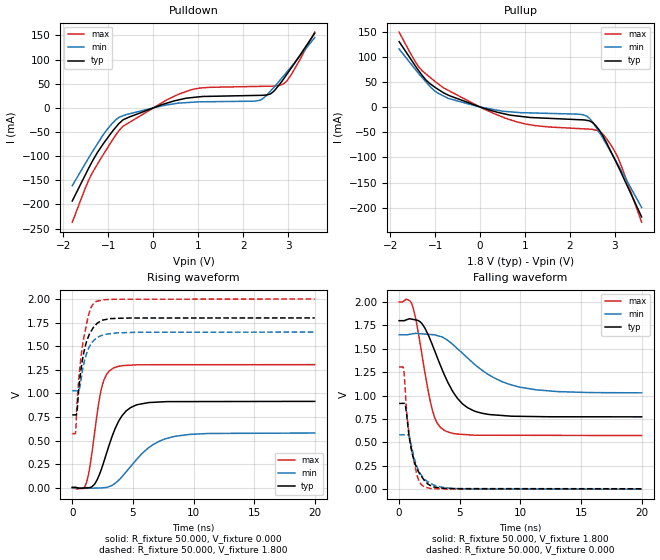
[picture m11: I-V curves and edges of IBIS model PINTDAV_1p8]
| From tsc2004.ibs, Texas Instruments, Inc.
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| Model 1.8 V PINTDAV
[Model]   PINTDAV_1p8
Model_type  Output
Polarity   Non-Inverting
Enable   Active-Low
Vmeas = 0.9
Vref = 0.9
Cref = 15pF
Rref = 50
|   typ   min   max
|   (nom PVT)   (Fast PVT)   (slow PVT)
|   Output High
C_comp   8.87322E-12   8.67118E-12   8.99669E-12
|   Output Low
|C_comp   8.83242E-12   8.51294E-12   9.03821E-12
| Where   nom PVT is  Nominal Process, 3.3V, 25C
|   Fast PVT is Strong Process, 3.6V, -40C
|   Slow PVT is Weak Process, 3.0V, 85C
|C_comp - from L-C Tank method, L = 1nH, peak frequency ~ 1.7GHz
[Voltage Range]   1.8   1.65   2
[Temperature Range]   30   88   -40
|Ambient Temperature Range 27   85   -40
[Pullup Reference]   1.8   1.65   2
[Pulldown Reference]   0   0   0
[Power Clamp Reference]   1.8   1.65   2
[GND Clamp Reference]   0   0   0
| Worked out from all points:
|   slope of the pulldown table from 0 to 0.27 V, typ, clamps not added: 30 ohm
|   slope of the pullup table from 0 to 0.27 V, typ, clamps not added: 35.3 ohm
|   falling waveform, R_fixture 50.000, V_fixture 1.800: 20-80 % time 2.19ns typ, 3.82ns min, 1.19ns max; typ from 1.8 V to 0.773 V
|   rising waveform, R_fixture 50.000, V_fixture 0.000: 20-80 % time 1.58ns typ, 2.67ns min, 896ps max; typ from 0.004 V to 0.915 V
|   rising waveform, R_fixture 50.000, V_fixture 1.800: 20-80 % time 817ps typ, 825ps min, 772ps max; typ from 0.773 V to 1.8 V
|   falling waveform, R_fixture 50.000, V_fixture 0.000: 20-80 % time 926ps typ, 1.03ns min, 772ps max; typ from 0.915 V to 0.004 V
[Pulldown]
|   Voltage   I(typ)   I(min)   I(max)
-1.8V     -192.8mA   -161.2mA   -236.8mA
-1.367V   -113.1mA   -93.03mA   -136.8mA
-929mV    -51.54mA   -34.05mA   -69.98mA
-672.1mV  -25.07mA   -16.42mA   -38.26mA
304.8mV   9.753mA    6.08mA     16.62mA
857.6mV   21.19mA    11.51mA    37.73mA
2.253V    25.62mA    13.81mA    44.22mA
2.436V    25.95mA    18.87mA    44.55mA
2.598V    28.47mA    33.64mA    44.83mA
2.8V      47.43mA    54.84mA    46.31mA
2.975V    69.69mA    74.32mA    55.61mA
3.595V    154.7mA    145.6mA    156.9mA
[Pullup]
|   Voltage   I(typ)   I(min)   I(max)
-1.8V     130mA      115.4mA    149.1mA
-1.281V   62.11mA    57.86mA    71.56mA
-1.017V   40.27mA    32.77mA    52.02mA
-704.3mV  23.56mA    17.18mA    33.06mA
24.07mV   -504.5uA   -278.9uA   -1.076mA
1.03V     -19.85mA   -11.4mA    -34.01mA
2.201V    -25.11mA   -14.15mA   -42.81mA
2.5V      -30.54mA   -29.5mA    -44.37mA
2.7V      -52.62mA   -57.02mA   -51.07mA
2.988V    -102.5mA   -101.6mA   -86.38mA
3.139V    -130.6mA   -125.7mA   -116.3mA
3.595V    -218.5mA   -199.7mA   -228.9mA
[Ramp]
R_load = 50
|   typ   min   max
dV/dt_r   0.561804/1.57452e-009  0.347932/2.64803e-009  0.782955/8.93072e-010
dV/dt_f   0.616385/2.18562e-009   0.37262/3.79469e-009  0.856164/1.19045e-009
[Falling Waveform]
R_fixture = 50.000
V_fixture = 1.800
V_fixture_min = 1.650
V_fixture_max = 2.000
C_fixture = 0.000
|  time   V(typ)   V(min)   V(max)
0s        1.8V       1.65V      2V
1.095ns   1.815V     1.659V     1.961V
1.91ns    1.764V     1.659V     1.413V
2.723ns   1.547V     1.651V     852.5mV
3.133ns   1.411V     1.641V     708.1mV
3.749ns   1.216V     1.611V     626.1mV
5.196ns   915.1mV    1.455V     585.3mV
6.838ns   810.9mV    1.271V     576.1mV
11.33ns   775.4mV    1.061V     575.1mV
20ns      772.7mV    1.029V     573.1mV
[Rising Waveform]
R_fixture = 50.000
V_fixture = 0.000
V_fixture_min = 0.000
V_fixture_max = 0.000
C_fixture = 0.000
|  time   V(typ)   V(min)   V(max)
0s        4.324mV    1.068uV    30.67nV
1.151ns   -1.527mV   -6.198mV   45.59mV
1.827ns   36.11mV    -4.034mV   568mV
2.411ns   200.4mV    -2.164mV   1.054V
2.816ns   361.1mV    3.376mV    1.199V
3.439ns   595.4mV    38.12mV    1.272V
4.804ns   849.1mV    223.4mV    1.299V
6.328ns   903mV      426.7mV    1.303V
8.303ns   912.9mV    540.5mV    1.304V
20ns      915.4mV    579.9mV    1.305V
[Rising Waveform]
R_fixture = 50.000
V_fixture = 1.800
V_fixture_min = 1.650
V_fixture_max = 2.000
C_fixture = 0.000
|  time   V(typ)   V(min)   V(max)
0s        772.7mV    1.029V     573.1mV
280.3ps   771.8mV    1.028V     597.8mV
398.1ps   814.7mV    1.027V     906.5mV
549.9ps   1.062V     1.036V     1.169V
739.7ps   1.273V     1.158V     1.408V
960.5ps   1.439V     1.319V     1.599V
1.471ns   1.642V     1.509V     1.885V
1.964ns   1.731V     1.583V     1.974V
4.572ns   1.799V     1.645V     1.999V
20ns      1.8V       1.65V      2V
[Falling Waveform]
R_fixture = 50.000
V_fixture = 0.000
V_fixture_min = 0.000
V_fixture_max = 0.000
C_fixture = 0.000
|  time   V(typ)   V(min)   V(max)
0s        915.4mV    579.9mV    1.305V
377ps     917mV      581.4mV    1.279V
548.5ps   868.7mV    582.1mV    956mV
763.5ps   626.6mV    574mV      649.5mV
1.045ns   400.5mV    444.1mV    412.1mV
1.342ns   262.8mV    287.8mV    221.4mV
1.661ns   171.9mV    185.9mV    82.54mV
2.069ns   94.61mV    111.8mV    23.78mV
4.292ns   7.356mV    7.798mV    1.198mV
20ns      4.324mV    1.068uV    13.14nV
